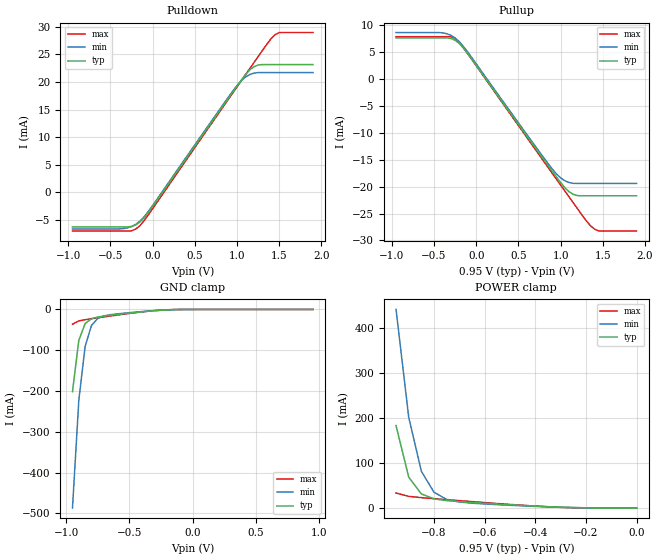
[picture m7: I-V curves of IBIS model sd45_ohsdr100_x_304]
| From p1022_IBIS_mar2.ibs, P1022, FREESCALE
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[Model]   sd45_ohsdr100_x_304
Model_type 3-state
Enable Active-High
Polarity Non-Inverting
|   TYP   MIN   MAX
C_comp   1.60pF   1.60pF   1.67pF
[Model Spec]
Vmeas   0.475   0.425   0.605
[Voltage Range]   0.95   0.85   1.21
[Temperature Range] 65   125   -40
[Driver Schedule]
| Model_Name  Rise_on_dly   Rise_off_dly   Fall_on_dly   Fall_off_dly
sd45_ohsdr100_x_30   0ps   NA   0ps   NA
sd45_ohsdr100_x_34   320ps   NA   320ps   NA
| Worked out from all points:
|   slope of the pulldown table from 0 to 0.142 V, typ, clamps not added: 45.6 ohm
|   slope of the pullup table from 0 to 0.142 V, typ, clamps not added: 45.5 ohm
|   GND clamp passes 1 mA (typ) near -0.19 V on its own axis
|   POWER clamp passes 1 mA (typ) near -0.25 V on its own axis
[Pullup]
|   Vout(V)   TYP   WCS   BCS
-950mV    7.673mA    8.666mA    7.886mA
-400mV    7.673mA    8.608mA    7.886mA
-250mV    7.224mA    7.649mA    7.542mA
-100mV    4.728mA    5.025mA    4.721mA
800mV     -14.94mA   -14.6mA    -15.28mA
1V        -19.23mA   -18.36mA   -19.69mA
1.1V      -20.94mA   -19.22mA   -21.89mA
1.15V     -21.42mA   -19.37mA   -22.99mA
1.3V      -21.69mA   -19.39mA   -26.25mA
1.4V      -21.69mA   -19.39mA   -27.87mA
1.5V      -21.69mA   -19.39mA   -28.26mA
1.9V      -21.69mA   -19.39mA   -28.26mA
[Pulldown]
|   Vout(V)   TYP   WCS   BCS
-950mV    -6.32mA    -6.677mA   -7.074mA
-350mV    -6.32mA    -6.625mA   -7.074mA
-250mV    -6.223mA   -6.253mA   -7.019mA
-150mV    -5.42mA    -5.26mA    -6.077mA
0V        -2.59mA    -2.42mA    -2.989mA
950mV     18.18mA    18.36mA    18.02mA
1.1V      21.33mA    20.89mA    21.32mA
1.2V      22.77mA    21.6mA     23.52mA
1.25V     23.08mA    21.7mA     24.61mA
1.45V     23.16mA    21.7mA     28.57mA
1.5V      23.16mA    21.7mA     28.97mA
1.9V      23.16mA    21.7mA     28.98mA
[GND Clamp]
|   Vout(V)   TYP   WCS   BCS
-950mV    -201.6mA   -486.5mA   -36.16mA
-900mV    -75.75mA   -222.9mA   -28.05mA
-850mV    -34.66mA   -90.59mA   -25.11mA
-800mV    -22.71mA   -39.37mA   -22.78mA
-750mV    -18.57mA   -21.91mA   -20.52mA
-700mV    -16.25mA   -15.71mA   -18.29mA
-650mV    -14.32mA   -12.88mA   -16.07mA
-400mV    -5.858mA   -5.175mA   -5.911mA
-200mV    -1.108mA   -1.072mA   -756.7uA
950mV     70.01uA    122.9uA    16.34uA
[POWER Clamp]
|   Vout(V)   TYP   WCS   BCS
-950mV    183.5mA    442.2mA    33.42mA
-900mV    68.86mA    202.2mA    25.88mA
-850mV    31.34mA    81.75mA    23.04mA
-800mV    20.35mA    35.06mA    20.76mA
-750mV    16.45mA    19.08mA    18.55mA
-700mV    14.22mA    13.35mA    16.36mA
-650mV    12.35mA    10.71mA    14.18mA
-300mV    1.805mA    1.559mA    1.409mA
0V        0A         0A         0A
[Ramp]
R_load=50.00
dV/dt_r  2.2428e-01/6.4141e-11  1.9173e-01/6.5657e-11  3.0370e-01/6.5055e-11
dV/dt_f  2.2428e-01/6.6042e-11  1.9173e-01/6.8481e-11  3.0372e-01/6.6195e-11
